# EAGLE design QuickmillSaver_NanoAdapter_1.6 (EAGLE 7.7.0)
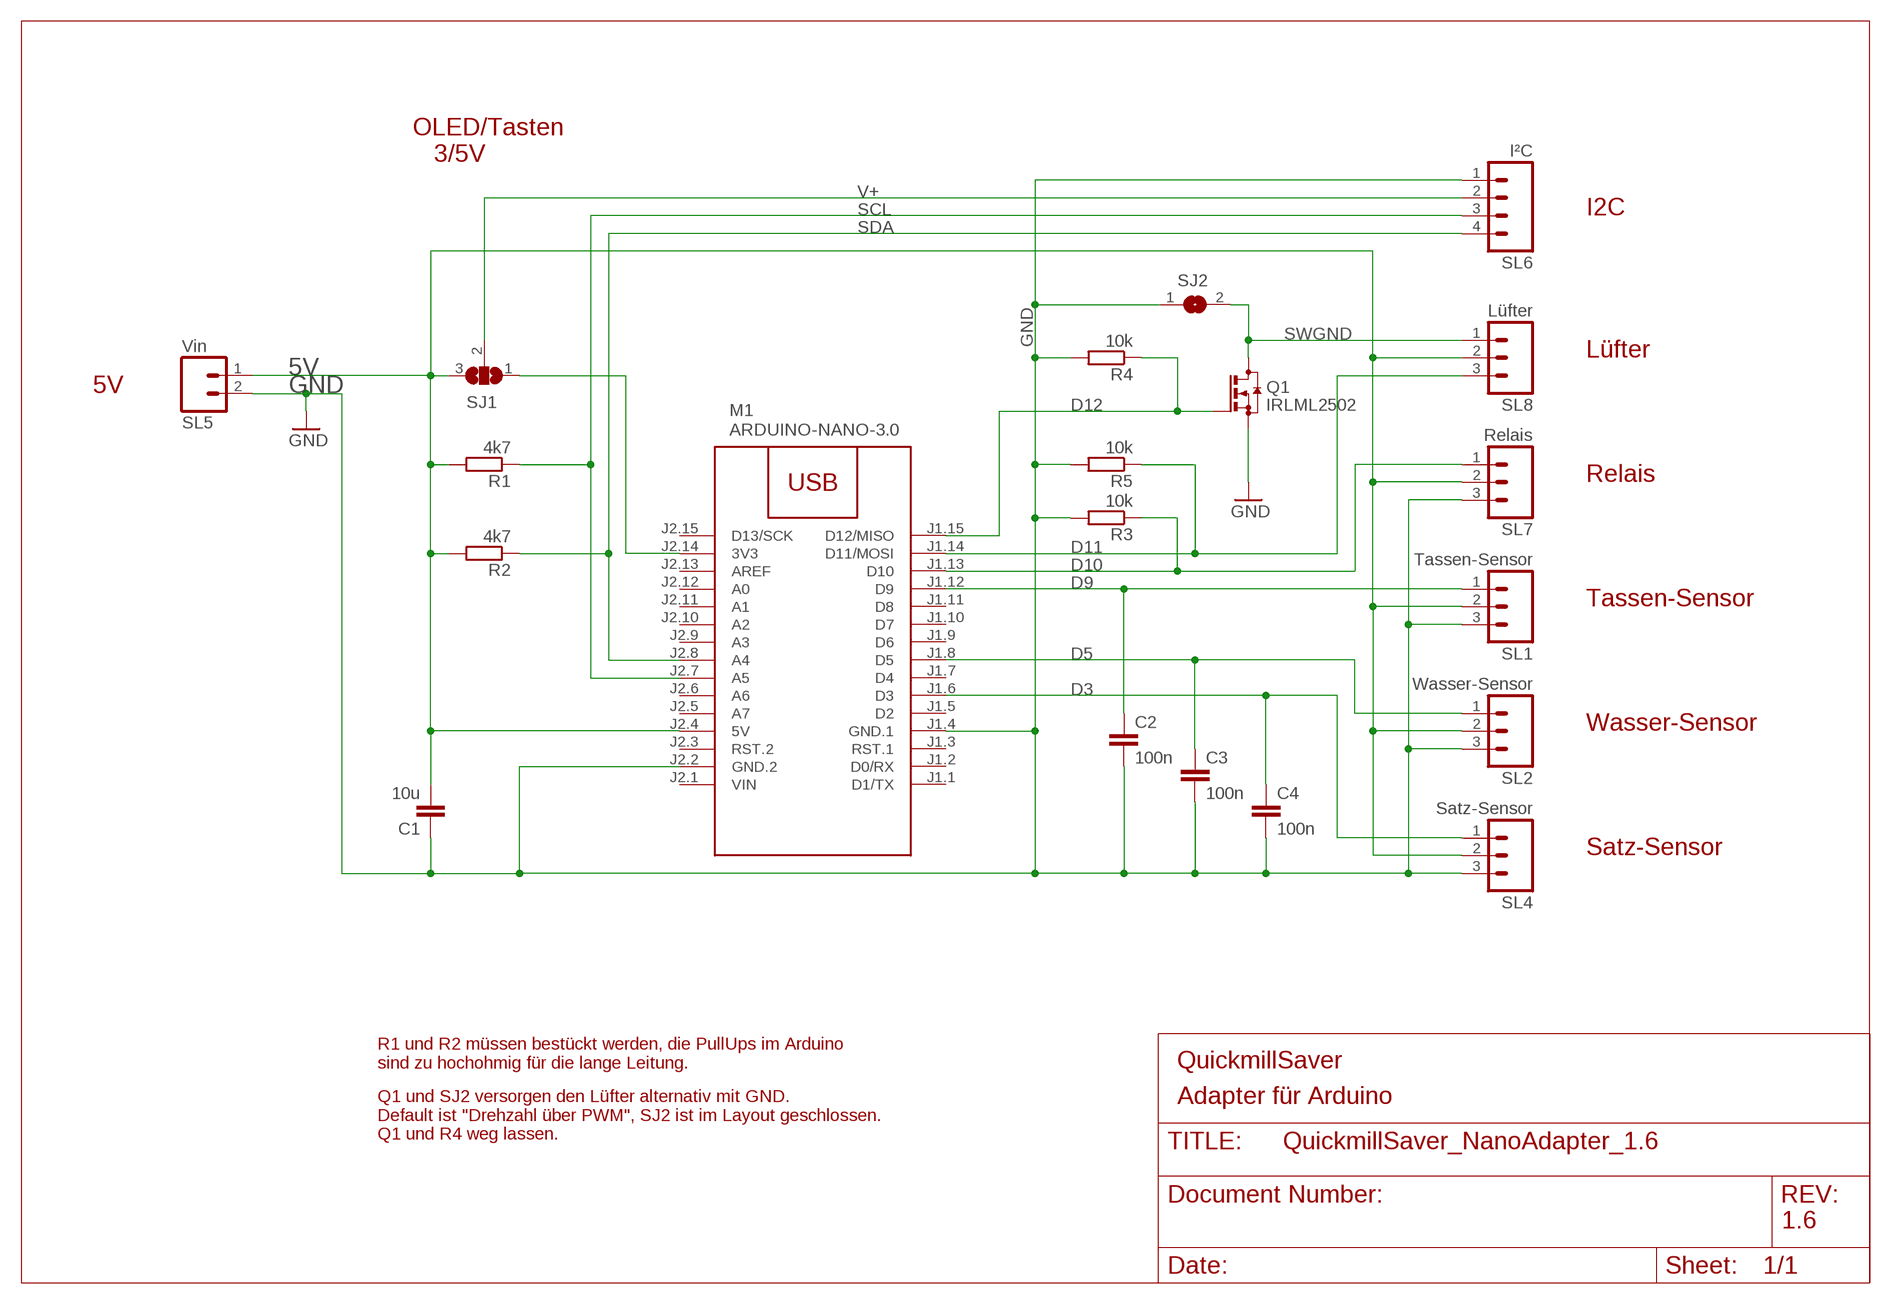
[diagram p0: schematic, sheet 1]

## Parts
C1  10u  C-EUC0805  [C0805]
C2  100n  C-EUC0603  [C0603]
C3  100n  C-EUC0603  [C0603]
C4  100n  C-EUC0603  [C0603]
M1  ARDUINO-NANO-3.0  [ARDUINO-NANO-3.0]
Q1  IRLML2502  BSS123  [SOT23]
R1  4k7  R-EU_R0603  [R0603]
R2  4k7  R-EU_R0603  [R0603]
R3  10k  R-EU_R0603  [R0603]
R4  10k  R-EU_R0603  [R0603]
R5  10k  R-EU_R0603  [R0603]
SJ1  SJ2WW  [SJ_2W]
SJ2  SJ  [SJ]
SL1  Tassen-Sensor  M03  [03P]
SL2  Wasser-Sensor  M03  [03P]
SL4  Satz-Sensor  M03  [03P]
SL5  Vin  M02  [02P]
SL6  I²C  M04  [04P]
SL7  Relais  M03  [03P]
SL8  Lüfter  M03  [03P]

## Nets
5V: C1.2 M1.J2.4(5V) R1.2 R2.2 SJ1.3 SL1.2 SL2.2 SL4.2 SL5.1 SL7.2 SL8.2
D3: C4.1 M1.J1.6(D3) SL4.1
D5: C3.1 M1.J1.8(D5) SL2.1
D9: C2.1 M1.J1.12(D9) SL1.1
D10: M1.J1.13(D10) R3.1 SL7.1
D11: M1.J1.14(D11/MOSI) R5.1 SL8.3
D12: M1.J1.15(D12/MISO) Q1.1(G) R4.1
GND: C1.1 C2.2 C3.2 C4.2 M1.J1.4(GND.1) M1.J2.2(GND.2) Q1.2(S) R3.2 R4.2 R5.2 SJ2.1 SL1.3 SL2.3 SL4.3 SL5.2 SL6.1 SL7.3
N$1: M1.J2.14(3V3) SJ1.1
SCL: M1.J2.7(A5) R1.1 SL6.3
SDA: M1.J2.8(A4) R2.1 SL6.4
SWGND: Q1.3(D) SJ2.2 SL8.1
V+: SJ1.2 SL6.2
Unconnected: M1.J1.1(D1/TX) M1.J1.2(D0/RX) M1.J1.3(RST.1) M1.J1.5(D2) M1.J1.7(D4) M1.J1.9(D6) M1.J1.10(D7) M1.J1.11(D8) M1.J2.3(RST.2) M1.J2.5(A7) M1.J2.6(A6) M1.J2.9(A3) M1.J2.10(A2) M1.J2.11(A1) M1.J2.12(A0) M1.J2.13(AREF) M1.J2.15(D13/SCK)

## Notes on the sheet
- OLED/Tasten
     3/5V
- I2C
- Lüfter
- 5V
- Relais
- Tassen-Sensor
- Wasser-Sensor
- Satz-Sensor
- R1 und R2 müssen bestückt werden, die PullUps im Arduino
  sind zu hochohmig für die lange Leitung.
- QuickmillSaver
- Adapter für Arduino
- Q1 und SJ2 versorgen den Lüfter alternativ mit GND.
  Default ist "Drehzahl über PWM", SJ2 ist im Layout geschlossen. 
  Q1 und R4 weg lassen.
- 1.6

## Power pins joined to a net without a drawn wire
VIN: M1.J2.1(VIN)

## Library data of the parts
C1-C4 = rcl:C-EU: CAPACITOR, European symbol
M1 = diy-modules:ARDUINO-NANO-3.0: Arduino Nano 3.0 and compatible devices More details available here: https://www.arduino.cc/en/Main/ArduinoBoardNano Click here to find device on ebay.com
Q1 = transistor-small-signal:BSS123: N-CHANNEL MOS FET
R1-R5 = rcl:R-EU_: RESISTOR, European symbol
SJ1 = jumper:SJ2W: SMD solder JUMPER
SJ2 = jumper:SJ: SMD solder JUMPER
SL1 SL2 SL4 SL7 SL8 = con-amp-quick:M03: AMP QUICK CONNECTOR
SL5 = con-amp-quick:M02: AMP QUICK CONNECTOR
SL6 = con-amp-quick:M04: AMP QUICK CONNECTOR

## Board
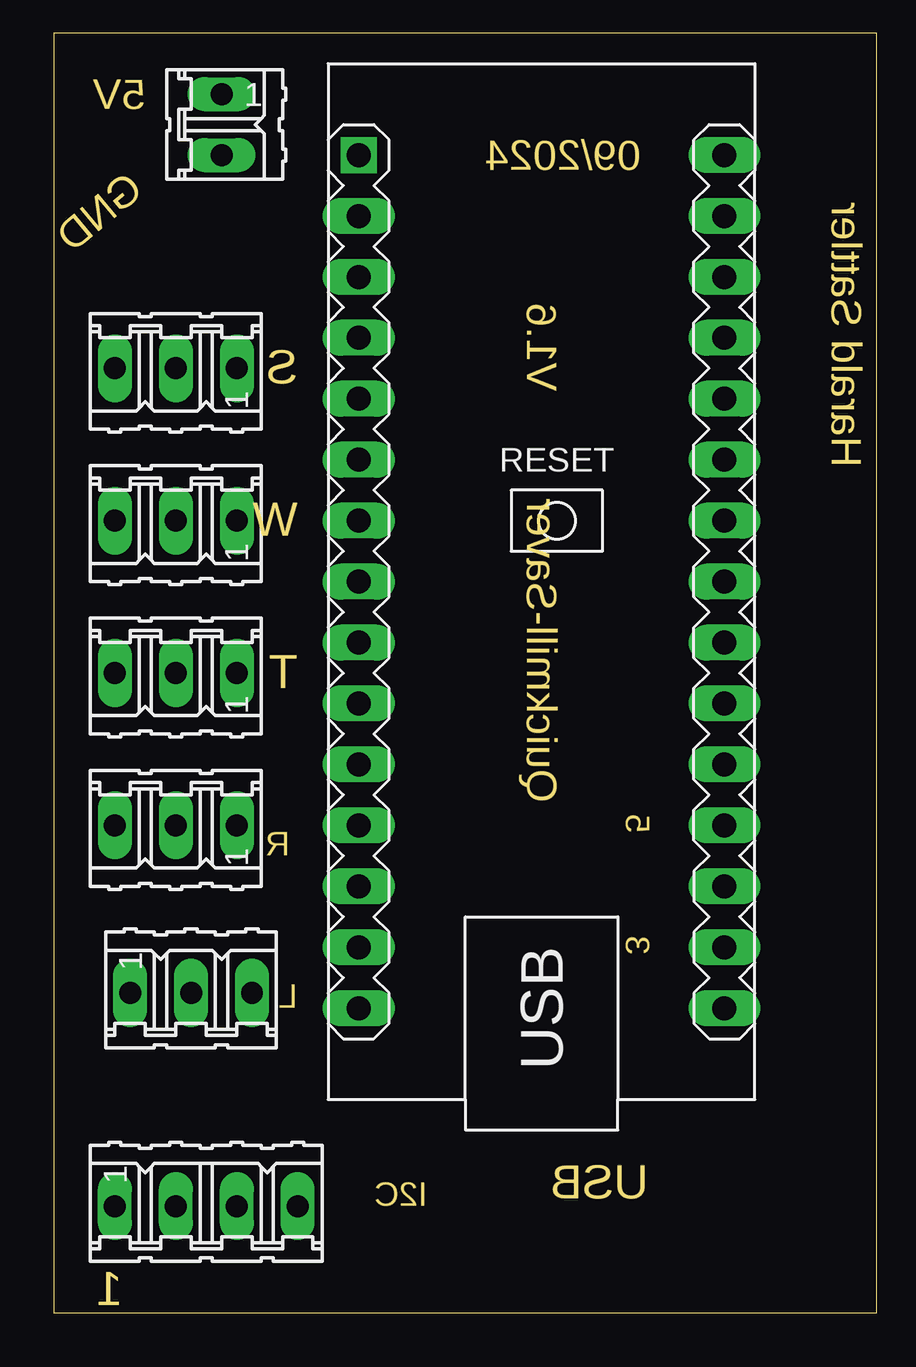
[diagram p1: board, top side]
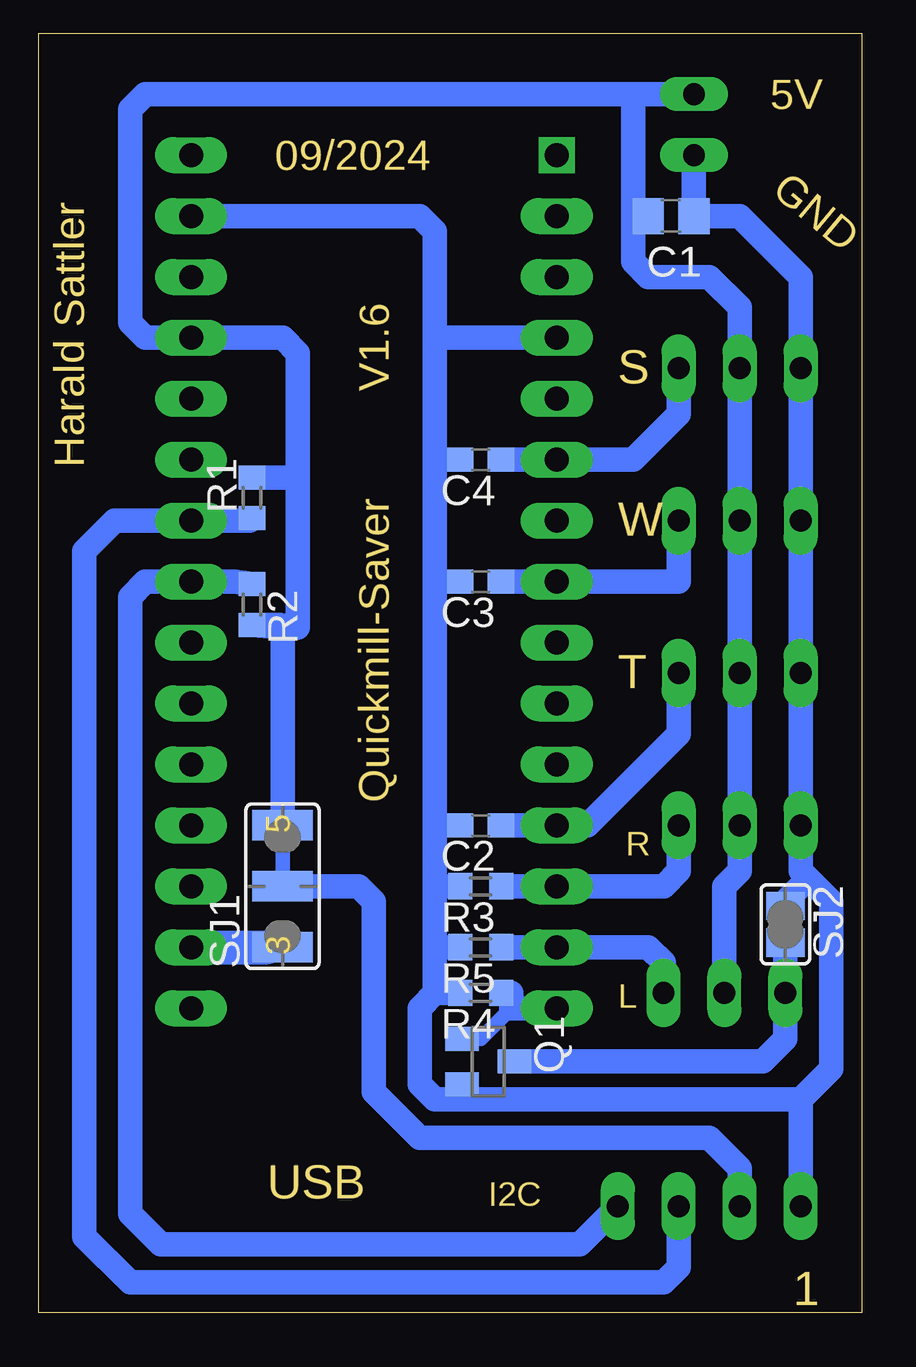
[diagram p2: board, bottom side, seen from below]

No outline drawn. Coordinates in mm, seen from the top.
Copper layers (1*16): Top 0.035mm / dielectric 1.5mm / Bottom 0.035mm
Design rules "default *": minimum track width 10mil, minimum drill 24mil, track to track 0.3mm, track to pad 0.3mm, pad to pad 0.3mm, via to via 0.3mm, smd to smd 0.3mm, copper to edge 40mil, drill to drill 8mil, minimum pad ring 10mil, minimum via ring 8mil, stop-mask expansion 4mil, vias tented up to drill 0mil, thermal gap 10mil
Milling: 4 lines

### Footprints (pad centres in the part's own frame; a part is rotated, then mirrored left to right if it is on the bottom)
C0805 = smd 1.3 x 1.5: 1 -0.95,0; 2 0.95,0
C0603 = smd 1.1 x 1: 1 -0.85,0; 2 0.85,0
ARDUINO-NANO-3.0 = drill 1 pad 1.27 square: J1.1 17.78,7.62 | drill 1 pad 1.27 long: J1.2 15.24,7.62; J1.3 12.7,7.62; J1.4 10.16,7.62; J1.5 7.62,7.62; J1.6 5.08,7.62; J1.7 2.54,7.62; J1.8 0,7.62; J1.9 -2.54,7.62; J1.10 -5.08,7.62; J1.11 -7.62,7.62; J1.12 -10.16,7.62; J1.13 -12.7,7.62; J1.14 -15.24,7.62; J1.15 -17.78,7.62; J2.1 17.78,-7.62; J2.2 15.24,-7.62; J2.3 12.7,-7.62; J2.4 10.16,-7.62; J2.5 7.62,-7.62; J2.6 5.08,-7.62; J2.7 2.54,-7.62; J2.8 0,-7.62; J2.9 -2.54,-7.62; J2.10 -5.08,-7.62; J2.11 -7.62,-7.62; J2.12 -10.16,-7.62; J2.13 -12.7,-7.62; J2.14 -15.24,-7.62; J2.15 -17.78,-7.62
SOT23 = smd 1 x 1.4: 1 -0.95,-1.1; 2 0.95,-1.1; 3 0,1.1
R0603 = smd 1 x 1.1: 1 -0.85,0; 2 0.85,0
SJ_2W = smd 1.27 x 2.54: 1 -2.54,0; 2 0,0; 3 2.54,0
SJ = smd 1.168 x 1.6: 1 -0.762,0; 2 0.762,0
03P = drill 0.914 long: 1 -2.54,0; 2 0,0; 3 2.54,0
02P = drill 0.914 long: 1 -1.27,0; 2 1.27,0
04P = drill 0.914 long: 1 -3.81,0; 2 -1.27,0; 3 1.27,0; 4 3.81,0

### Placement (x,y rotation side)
C1  7.94,45.72 180 bottom
C2  15.88,20.32 180 bottom
C3  15.88,30.48 180 bottom
C4  15.88,35.56 180 bottom
M1  20.32,30.48 90 top
Q1  15.56,10.48 270 bottom
R1  25.4,33.97 90 bottom
R2  25.4,29.53 270 bottom
R3  15.88,17.78 180 bottom
R4  15.88,13.34 180 bottom
R5  15.88,15.24 180 bottom
SJ1  24.13,17.78 90 bottom
SJ2  3.17,16.19 270 bottom
SL1  5.08,26.67 180 top
SL2  5.08,33.02 180 top
SL4  5.08,39.37 180 top
SL5  6.99,49.53 270 top
SL6  6.35,4.45 0 top
SL7  5.08,20.32 180 top
SL8  5.71,13.34 0 top

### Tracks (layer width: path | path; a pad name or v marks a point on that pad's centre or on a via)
5V
  Bottom 0.61: SJ1.3 24.13,17.78
  Bottom 1.016: 23.5,34.92 23.5,40.01 24.13,40.64 M1.J2.4 29.84,40.64 30.48,41.27 30.48,50.16 29.84,50.8 9.53,50.8 | 23.5,34.92 23.5,28.57 24.23,28.68 R2.2 24.13,28.57 SJ1.3 | R1.2 23.6,34.82 23.5,34.92 | SL5.1 9.53,50.8 | 9.53,45.72 9.53,43.81 8.89,43.18 6.35,43.18 5.08,41.91 SL4.2 SL2.2 SL1.2 SL7.2 5.08,18.41 5.71,17.78 SL8.2 | 9.53,45.72 9.53,50.8 | C1.2 9.53,45.72
D3
  Bottom 1.016: SL4.1 7.62,37.47 9.53,35.56 M1.J1.6 C4.1
D5
  Bottom 1.016: SL2.1 7.62,30.48 M1.J1.8 C3.1
D9
  Bottom 1.016: SL1.1 7.62,24.13 11.43,20.32 M1.J1.12 C2.1
D10
  Bottom 1.016: SL7.1 7.62,18.41 8.26,17.78 M1.J1.13 R3.1
D11
  Bottom 1.016: SL8.3 8.26,14.61 8.89,15.24 M1.J1.14 R5.1
D12
  Bottom 0.61: 16.51,11.43 15.88,11.43 14.61,12.7
  Bottom 1.016: R4.1 14.61,13.34 14.61,12.7 M1.J1.15 | Q1.1 16.51,11.43
GND
  Bottom 0.406: SJ2.1 3.17,15.24
  Bottom 1.016: 17.78,40.64 17.78,45.09 18.41,45.72 M1.J2.2 | SL5.2 C1.1 | SL6.1 2.54,8.89 | 2.54,8.89 1.27,10.16 1.27,17.14 2.22,18.1 | 2.22,18.1 2.54,18.41 SL7.3 SL1.3 SL2.3 SL4.3 2.54,43.18 5.08,45.72 C1.1 | M1.J1.4 17.78,40.64 | 17.78,40.64 17.78,35.56 | 17.78,35.56 17.78,30.48 | 17.78,30.48 17.78,20.32 | 17.78,20.32 17.78,17.78 | 17.78,17.78 17.78,15.24 | 17.78,15.24 17.78,13.34 | 16.51,8.89 17.78,8.89 18.41,9.53 18.41,12.7 17.78,13.34 | 16.51,8.89 2.54,8.89 | C3.2 17.78,30.48 | C4.2 17.78,35.56 | C2.2 17.78,20.32 | C1.1 | R3.2 17.78,17.78 | R5.2 17.78,15.24 | R4.2 17.78,13.34 | Q1.2 16.66,9.04 16.51,8.89 | SJ2.1 3.17,17.14 2.22,18.1
N$1
  Bottom 1.016: 24.77,15.24 SJ1.1
  Bottom 1.422: M1.J2.14 24.77,15.24
SCL
  Bottom 1.016: R1.1 25.5,33.02 M1.J2.7 31.11,33.02 32.38,31.75 32.38,3.17 30.48,1.27 8.26,1.27 7.62,1.91 SL6.3
SDA
  Bottom 1.016: R2.1 26.14,30.48 M1.J2.8 29.84,30.48 30.48,29.84 30.48,4.13 29.21,2.86 11.75,2.86 SL6.4
SWGND
  Bottom 1.016: Q1.3 4.13,10.48 3.17,11.43 SL8.1 SJ2.2
V+
  Bottom 1.016: SL6.2 5.08,6.03 6.35,7.3 18.41,7.3 20.32,9.21 20.32,17.14 20.95,17.78 SJ1.2

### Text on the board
Milling: 5V | 09/2024 | GND | S | V1.6 | Harald Sattler | W | T | Quickmill-Saver | 5 | R | 3 | L | USB | I2C | 1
